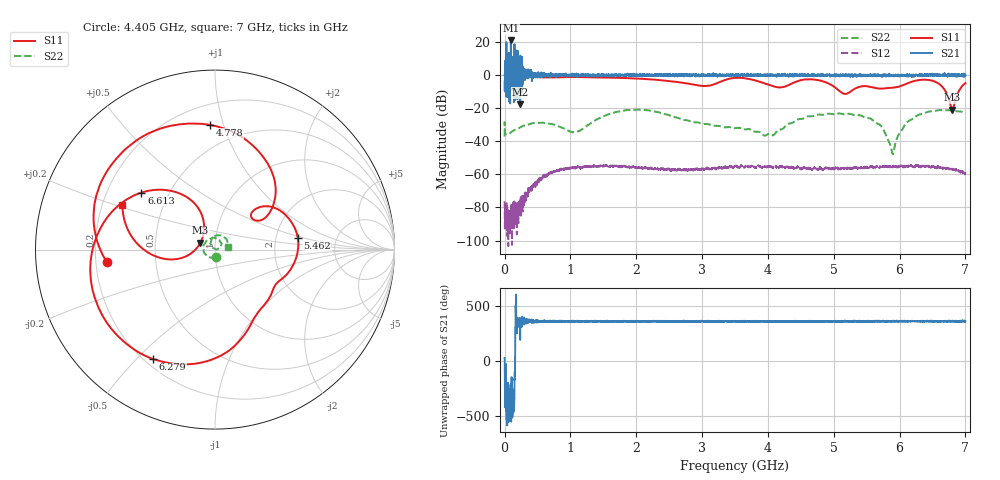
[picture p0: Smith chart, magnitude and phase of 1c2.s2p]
!Keysight Technologies,N5232A,MY52221221,A.10.65.11
!Date: Wednesday, October 16, 2024 12:01:48
!Correction: S11(Full 2 Port(1,4))
!S41(Full 2 Port(1,4))
!S14(Full 2 Port(1,4))
!S44(Full 2 Port(1,4))
!S2P File: Measurements: S11, S41, S14, S44:
# Hz S  RI  R 50
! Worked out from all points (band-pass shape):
!   4001 points, 300 kHz to 7 GHz, reference 50 ohm
!   highest |S21| = 20.95 dB at 94.8 MHz (marker M1); lowest = -17.7 dB at 236.5 MHz (marker M2)
!   |S21| within 3 dB of the highest: 26.39 MHz to 26.73 MHz (340.4 kHz wide, 1.28 % of centre); 94.51 MHz to 95.09 MHz (585.7 kHz wide, 0.618 % of centre)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
!   lowest |S11| = -20.9 dB at 6.802 GHz (marker M3), VSWR 1.20, Z = 42.4 + j3.35 ohm
!   |S11| at or under -10 dB: 5.1 GHz to 5.254 GHz (154.1 MHz wide, 2.98 % of centre); 6.702 GHz to 6.897 GHz (195.1 MHz wide, 2.87 % of centre)
!   |S22| runs from -47.7 to -20.8 dB; largest |S21 - S12| = 11
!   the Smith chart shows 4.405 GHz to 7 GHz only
!   S11 on the Smith chart (normalised r, x): 4.405 GHz: 0.25, -0.05; 4.778 GHz: 0.34, +0.91; 5.462 GHz: 2.65, +0.45; 6.279 GHz: 0.23, -0.56; 6.613 GHz: 0.35, +0.30; 7 GHz: 0.29, +0.21
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300000  -0.9955 -0.0114  0.5628 0.283  6.28e-05 0.00014  -0.012 -0.00721
3.704842e7  -0.9876 0.1257  -0.0481 -0.4173  8.88e-06 -5.2e-05  -0.0151 0.00611
9.479595e7  -0.9401 0.3119  11.13 0.8446  2.56e-05 2.45e-05  -0.011 0.0148
1.087954e8  -0.9232 0.3561  0.174 0.9777  5.99e-06 3.09e-05  -0.00995 0.0166
1.40294e8  -0.8758 0.4464  0.6346 0.4957  -4.61e-05 6.03e-05  -0.00734 0.02
2.365399e8  -0.6802 0.6817  -0.1282 -0.0262  2.09e-05 6.17e-05  0.00564 0.0256
6.75771e8  0.3942 0.7485  1.017 0.0327  8.4e-05 -0.001  0.0308 -0.0142
1.1675e9  0.8238 -0.2872  0.9465 -0.0161  5.6e-05 0.00165  -0.0193 0.0115
1.667979e9  -0.1799 -0.8133  1.019 -0.0283  0.000396 -0.00183  0.0721 0.0173
2.3347e9  -0.5676 0.4331  0.9653 0.0177  0.000408 0.00143  -0.0376 -0.066
3.228912e9  0.5104 0.2576  0.9525 0.0506  -0.00151 -0.000171  0.0268 -0.0117
3.50015e9  0.7026 -0.435  0.9624 0.0229  -0.0005 0.00174  -0.00948 -0.0229
3.871134e9  -0.2854 -0.5689  1.033 -0.0352  0.00174 -0.000415  -0.0117 0.0153
4.404861e9  -0.6035 -0.0665  1.071 0.03  -0.00154 -0.000307  0.00343 -0.0394
4.66735e9  -0.3774 0.6439  1.016 -0.0395  -0.000571 0.00134  -0.0446 -0.0356
4.777595e9  -0.0253 0.6942  1.011 0.0479  0.000129 0.0015  -0.0624 -0.0161
5.461816e9  0.461 0.0667  1.033 -0.0222  -0.000586 -0.00157  0.0286 0.0456
5.83455e9  0.2927 -0.2847  0.9316 -0.0101  -0.00111 0.00137  0.01 0.00028
6.279031e9  -0.3441 -0.6101  0.9836 0.0241  0.00174 -0.000499  -0.0188 0.0588
6.613267e9  -0.4102 0.3176  0.9914 -0.0355  -0.00109 -0.00111  0.0387 0.0787
6.802258e9  -0.081 0.0392  1.007 0.0416  -0.00127 0.000612  0.0664 0.0532
7e9  -0.5158 0.2459  0.9797 0.0121  0.000395 0.001  0.07 0.0142
